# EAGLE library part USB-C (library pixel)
USB Type-C USB 2.0 Connector
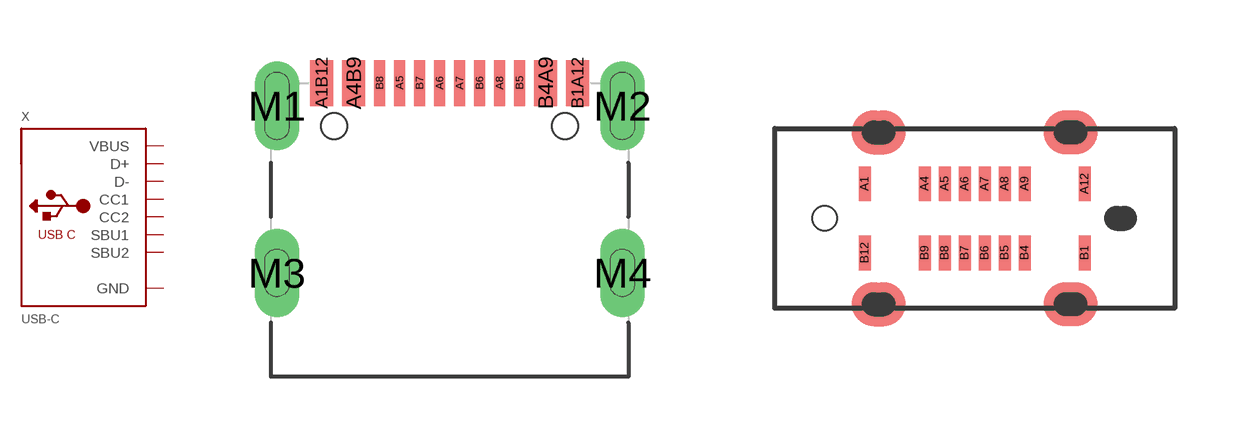
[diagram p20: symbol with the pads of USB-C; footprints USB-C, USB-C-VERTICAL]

Designator prefix X

## USB-C  [USB-C]
A1B12  GND  pwr
A4B9  VBUS  pwr
A5  CC1
A6  D+
A7  D-
A8  SBU1
B1A12  GND  pwr
B4A9  VBUS  pwr
B5  CC2
B6  D+
B7  D-
B8  SBU2
M1  GND  pwr
M2  GND  pwr
M3  GND  pwr
M4  GND  pwr

## USB-CVERTICAL  [USB-C-VERTICAL]
A1  GND  pwr
A4  VBUS  pwr
A5  CC1
A6  D+
A7  D-
A8  SBU1
A9  VBUS  pwr
A12  GND  pwr
B1  GND  pwr
B4  VBUS  pwr
B5  CC2
B6  D+
B7  D-
B8  SBU2
B9  VBUS  pwr
B12  GND  pwr

## Footprint USB-C (pad centres in mm)
smd 0.575 x 1.15: A1B12 -3.2,3.545; A4B9 -2.4,3.545; B1A12 3.2,3.545; B4A9 2.4,3.545
smd 0.275 x 1.15: A5 -1.25,3.545; A6 -0.25,3.545; A7 0.25,3.545; A8 1.25,3.545; B5 1.75,3.545; B6 0.75,3.545; B7 -0.75,3.545; B8 -1.75,3.545
drill 0.6 pad 1 long: M1 -4.32,2.97; M2 4.32,2.97; M3 -4.32,-1.21; M4 4.32,-1.21
hole 0.65 at 2.89,2.47
hole 0.65 at -2.89,2.47

## Footprint USB-C-VERTICAL (pad centres in mm)
smd 0.3 x 0.87: A1 -2.75,0.865; A4 -1.25,0.865; A5 -0.75,0.865; A6 -0.25,0.865; A7 0.25,0.865; A8 0.75,0.865; A9 1.25,0.865; A12 2.75,0.865; B1 2.75,-0.865; B4 1.25,-0.865; B5 0.75,-0.865; B6 0.25,-0.865; B7 -0.25,-0.865; B8 -0.75,-0.865; B9 -1.25,-0.865; B12 -2.75,-0.865
hole 0.62 at -3.75,0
